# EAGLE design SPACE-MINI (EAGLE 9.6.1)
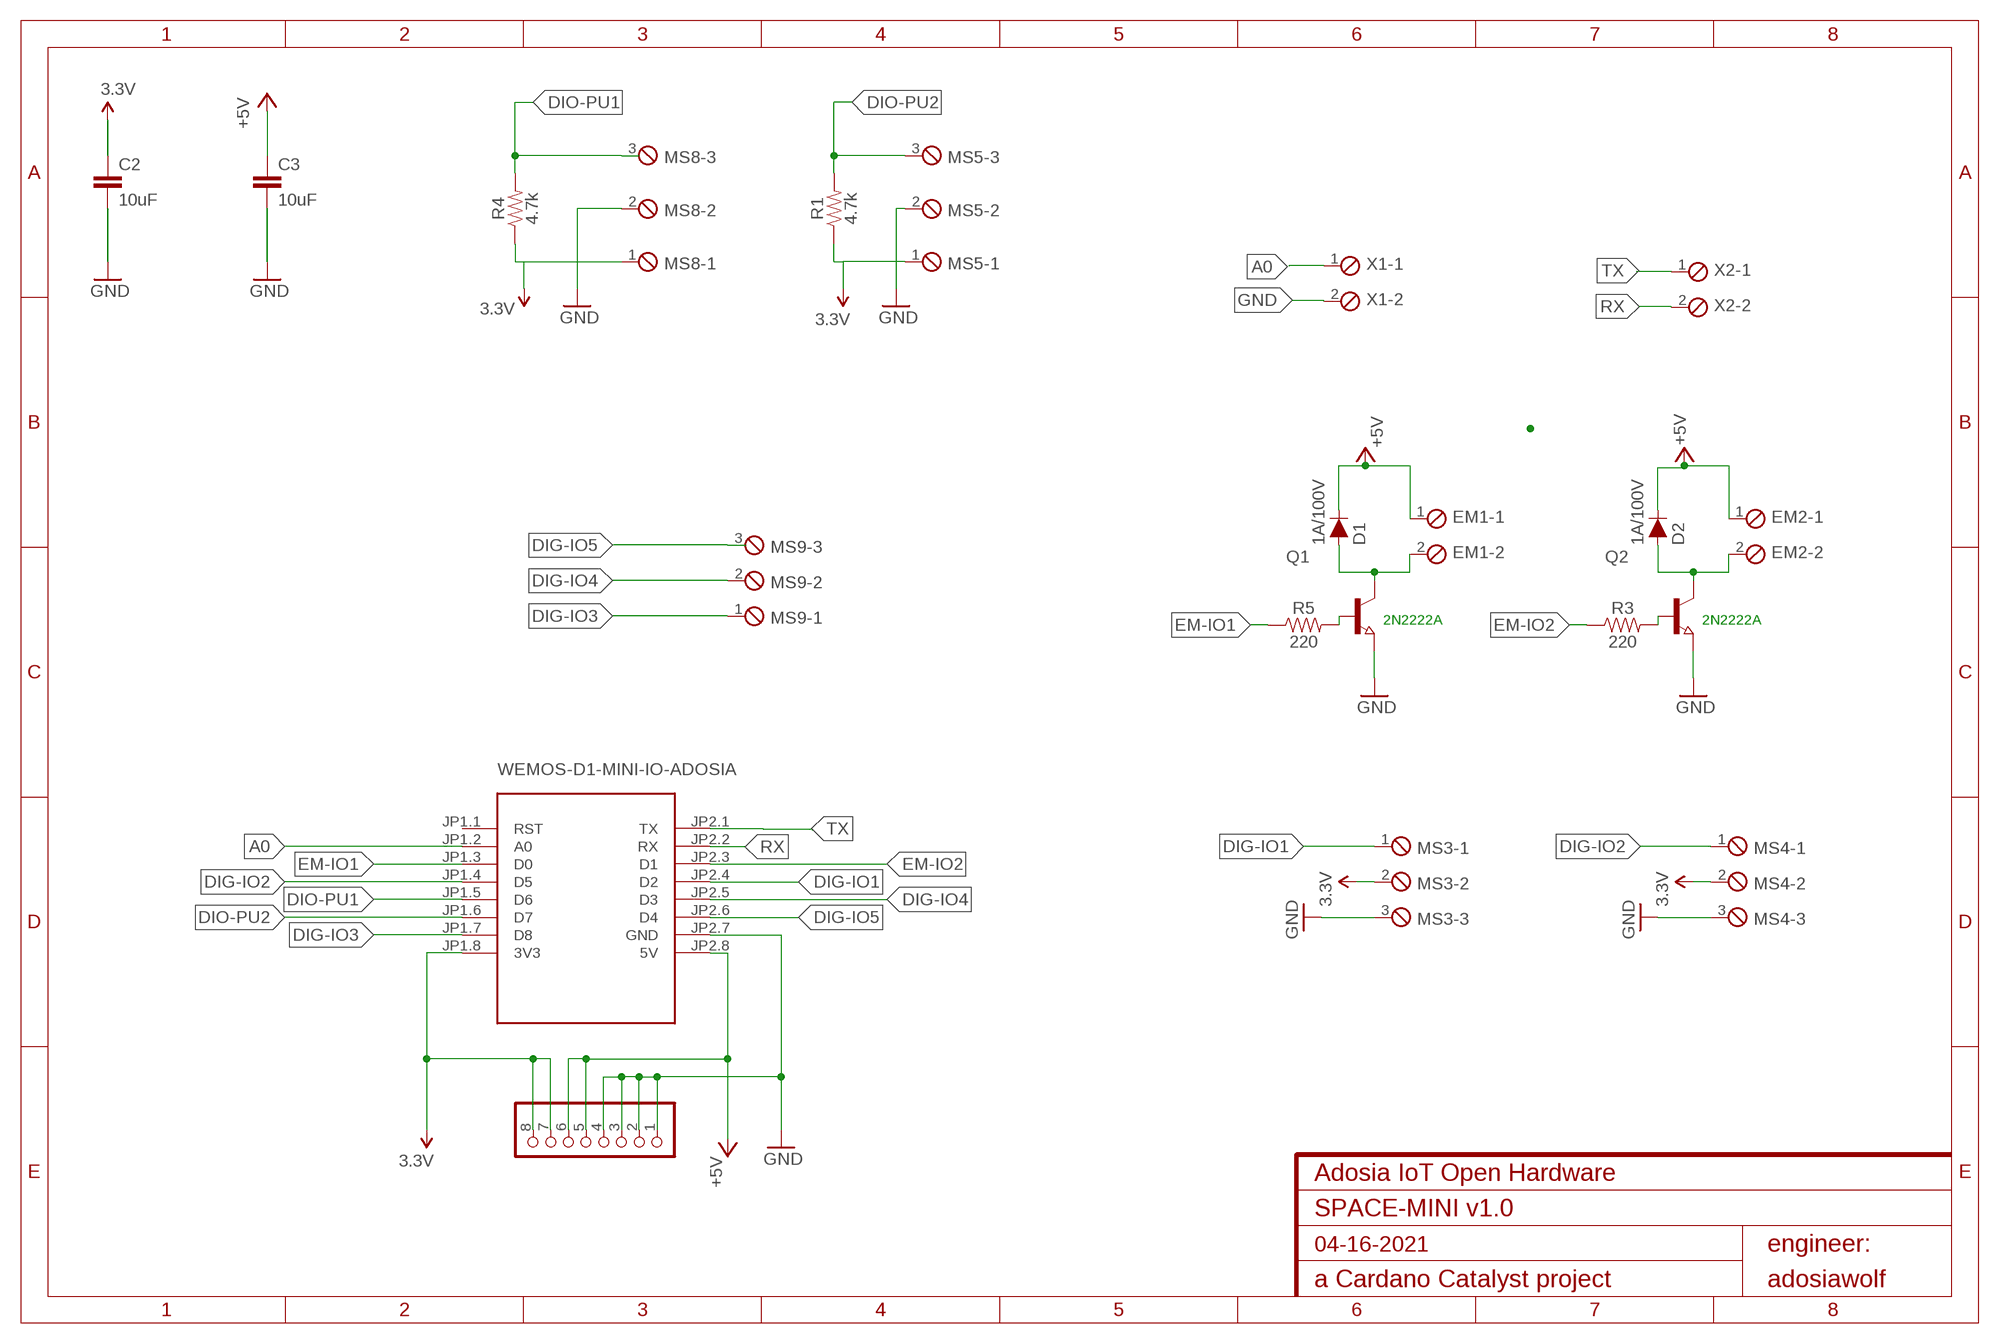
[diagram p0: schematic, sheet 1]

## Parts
C2  10uF  10UF-6.3V-20%(0603)  [0603-CAP@1]
C3  10uF  10UF-6.3V-20%(0603)  [0603-CAP@1]
D1  1A/100V  DIODE-BAS16J  [SOD-323]
D2  1A/100V  DIODE-BAS16J  [SOD-323]
EM1  MPT2  [2POL254]
EM2  MPT2  [2POL254]
JP1  PINHD-1X8/90  [1X08/90]
MS3  MPT3  [3POL254]
MS4  MPT3  [3POL254]
MS5  MPT3  [3POL254]
MS8  MPT3  [3POL254]
MS9  MPT3  [3POL254]
Q1  NPN-TRANSISTOR_SOT23  [SOT23]
Q2  NPN-TRANSISTOR_SOT23  [SOT23]
R1  4.7k  4.7KOHM-0603-1/10W-1%  [0603]
R3  220  220OHM-0603-1/10W-1%  [0603]
R4  4.7k  4.7KOHM-0603-1/10W-1%  [0603]
R5  220  220OHM-0603-1/10W-1%  [0603]
U$1  WEMOS-D1-MINI-IO-ADOSIA  [WEMOS-D1-MINI-SHIELD]
X1  MPT2  [2POL254]
X2  MPT2  [2POL254]

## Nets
3.3V: C2.1 JP1.7 JP1.8 MS3.2 MS4.2 MS5.1 MS8.1 R1.1 R4.1 U$1.JP1.8(3V3)
+5V: C3.1 D1.C D2.C EM1.1 EM2.1 JP1.5 JP1.6 U$1.JP2.8(5V)
A0: U$1.JP1.2(A0) X1.1
DIG-IO1: MS3.1 U$1.JP2.4(D2)
DIG-IO2: MS4.1 U$1.JP1.4(D5)
DIG-IO3: MS9.1 U$1.JP1.7(D8)
DIG-IO4: MS9.2 U$1.JP2.5(D3)
DIG-IO5: MS9.3 U$1.JP2.6(D4)
DIO-PU1: MS8.3 R4.2 U$1.JP1.5(D6)
DIO-PU2: MS5.3 R1.2 U$1.JP1.6(D7)
EM-IO1: R5.1 U$1.JP1.3(D0)
EM-IO2: R3.1 U$1.JP2.3(D1)
GND: C2.2 C3.2 JP1.1 JP1.2 JP1.3 JP1.4 MS3.3 MS4.3 MS5.2 MS8.2 Q1.2(E) Q2.2(E) U$1.JP2.7(GND) X1.2
N$2: Q2.1(B) R3.2
N$3: Q1.1(B) R5.2
N$4: D2.A EM2.2 Q2.3(C)
N$6: D1.A EM1.2 Q1.3(C)
RX: U$1.JP2.2(RX) X2.2
TX: U$1.JP2.1(TX) X2.1
Unconnected: U$1.JP1.1(RST)

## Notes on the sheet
- 2N2222A | 2N2222A

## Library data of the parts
C2 C3 = SparkFun-Capacitors:10UF-6.3V-20%(0603): CAP-11015; PROD_ID: CAP-11015
D1 D2 = SparkFun-DiscreteSemi:DIODE: Diode; PROD_ID: DIO-09646; VALUE: 250mA/100V
EM1 EM2 X1 X2 = con-phoenix-254:MPT2: PHOENIX CONNECTOR; OC_FARNELL: unknown; OC_NEWARK: unknown
JP1 = pinhead:PINHD-1X8: PIN HEADER
MS3-MS5 MS8 MS9 = con-phoenix-254:MPT3: PHOENIX CONNECTOR; OC_FARNELL: unknown; OC_NEWARK: unknown
Q1 Q2 = semicon-smd-ipc:NPN-TRANSISTOR_: NPN TRANSISTOR
R1 R4 = SparkFun-Resistors:4.7KOHM: 4.7kΩ resistor; PROD_ID: RES-07857
R3 R5 = SparkFun-Resistors:220OHM: 220Ω resistor; PROD_ID: RES-07861
U$1 = diy-modules:WEMOS-D1-MINI-IO-ADOSIA: Template for WEMOS D1 mini compatible shields NOTICE: This is a template only. You can use it as a base to create symbols for WEMOS D1 mini compatible shields. Official list of available shields can be found here: https://www.wemos.cc/D1-mini-Shields

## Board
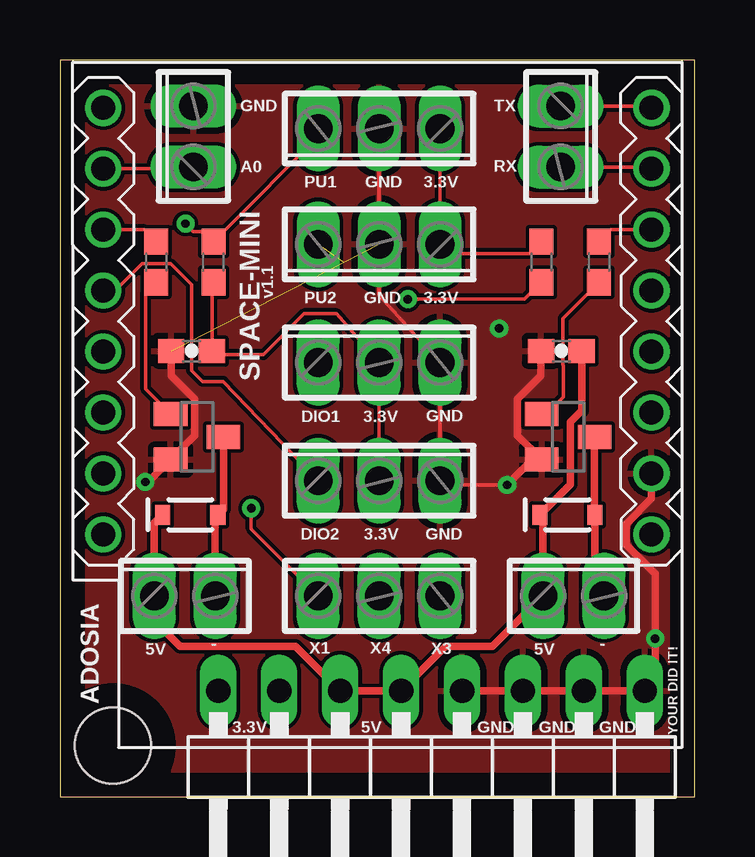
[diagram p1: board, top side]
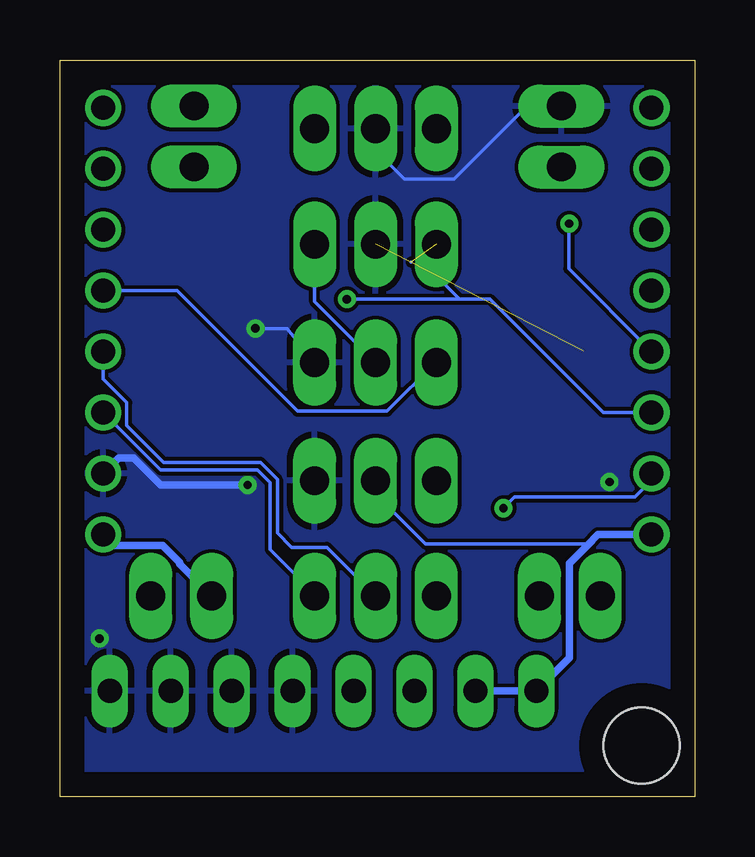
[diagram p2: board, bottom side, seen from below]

Size 26.47 x 30.72 mm. Coordinates in mm from the lower left corner, seen from the top.
Outline: 0,0 26.47,0 26.47,30.72 0,30.72 0,0
Copper layers (1*16): Top 0.035mm / dielectric 1.5mm / Bottom 0.035mm
Design rules "default": minimum track width 6mil, minimum drill 0.35mm, track to track 6mil, track to pad 6mil, pad to pad 6mil, via to via 6mil, smd to smd 6mil, copper to edge 40mil, drill to drill 6mil, minimum pad ring 10mil, minimum via ring 8mil, stop-mask expansion 4mil, vias tented up to drill 0mil, thermal gap 10mil
Holes 3.17 mm at 2.21,2.13

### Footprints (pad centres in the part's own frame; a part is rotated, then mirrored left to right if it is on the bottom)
0603-CAP@1 = smd 1.1 x 1: 1 -0.85,0; 2 0.85,0
SOD-323 = smd 0.63 x 0.83: A 1.15,0; C -1.15,0
2POL254 = drill 1.2 long: 1 -1.27,0; 2 1.27,0
1X08/90 = drill 1.016 long: 1 -8.89,-3.81; 2 -6.35,-3.81; 3 -3.81,-3.81; 4 -1.27,-3.81; 5 1.27,-3.81; 6 3.81,-3.81; 7 6.35,-3.81; 8 8.89,-3.81
3POL254 = drill 1.2 long: 1 -2.54,0; 2 0,0; 3 2.54,0
SOT23 = smd 1 x 1.4: 1 -0.95,-1.1; 2 0.95,-1.1; 3 0,1.1
0603 = smd 1.1 x 1: 1 -0.85,0; 2 0.85,0
WEMOS-D1-MINI-SHIELD = drill 1: JP1.1 -11.43,12.065; JP1.2 -11.43,9.525; JP1.3 -11.43,6.985; JP1.4 -11.43,4.445; JP1.5 -11.43,1.905; JP1.6 -11.43,-0.635; JP1.7 -11.43,-3.175; JP1.8 -11.43,-5.715; JP2.1 11.43,12.065; JP2.2 11.43,9.525; JP2.3 11.43,6.985; JP2.4 11.43,4.445; JP2.5 11.43,1.905; JP2.6 11.43,-0.635; JP2.7 11.43,-3.175; JP2.8 11.43,-5.715

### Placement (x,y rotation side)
C2  5.49,18.59 180 top
C3  20.9,18.59 180 top
D1  5.44,11.76 0 top
D2  21.16,11.76 0 top
EM1  5.21,8.38 0 top
EM2  21.41,8.38 0 top
JP1  15.49,0.61 180 top
MS3  13.31,18.11 0 top
MS4  13.31,13.18 0 top
MS5  13.31,23.04 180 top
MS8  13.31,27.86 180 top
MS9  13.31,8.38 0 top
Q1  5.71,15.01 270 top
Q2  21.18,15.01 270 top
R1  20.07,22.3 270 top
R3  22.48,22.3 270 top
R4  6.4,22.3 90 top
R5  4.01,22.3 270 top
U$1  13.23,16.66 0 top
X1  5.56,27.53 90 top
X2  20.88,27.53 270 top

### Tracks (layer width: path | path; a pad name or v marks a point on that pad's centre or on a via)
3.3V
  Top 0.152: R4.1 6.34,21.39 C2.1 6.49,18.44 8.48,18.44 10.19,20.14 11.53,20.14 MS3.2 MS4.2 | MS8.1 MS5.1 16.51,22.66 19.57,22.66 R1.1
  Bottom 0.152: JP1.7 9.45,4.42 | MS5.1 15.85,20.65 MS3.2 | MS4.2 13.31,12.62 11.23,10.54 4.5,10.54 4.46,10.51
  Bottom 0.305: U$1.JP1.8 2.39,10.95 2.39,10.94 4.03,10.94 4.46,10.51 5.23,9.74 5.23,5.79 JP1.8 JP1.7
+5V
  Top 0.305: D1.C 3.94,11.41 EM1.1 3.94,7.34 5,6.27 9.83,6.27 JP1.6 JP1.5 16.08,6.28 18.04,6.28 EM2.1 20.14,11.63 D2.C 21.28,13.03 21.28,15.64 21.75,16.11 C3.1
  Bottom 0.305: U$1.JP2.8 24.2,10.49 22.18,10.49 21.48,9.78 21.48,9.72 EM2.1
A0
  Top 0.152: U$1.JP1.2 5.49,26.19 X1.1
DIG-IO1
  Bottom 0.152: U$1.JP2.4 21.59,21.11 16.56,16.08 12.83,16.08 10.77,18.14 MS3.1
DIG-IO2
  Top 0.152: MS4.1 6.81,17.32 5.94,17.32 5.49,17.78 5.49,21.35 4.61,22.23 3.42,22.23 2.3,21.11 U$1.JP1.4
DIG-IO3  (via drill 0.35)
  Top 0.152: MS9.1 7.98,11.18 v7.98,12.04
  Bottom 0.152: v7.98,12.04 7.52,12.5 2.49,12.5 1.8,13.18 U$1.JP1.7
DIG-IO4
  Bottom 0.152: U$1.JP2.5 24.66,17.42 23.68,16.43 23.68,15.48 22.15,13.94 18.11,13.94 17.4,13.23 17.4,11 16.81,10.41 15.34,10.41 MS9.2
DIG-IO5
  Bottom 0.152: U$1.JP2.6 22.28,13.64 18.24,13.64 17.7,13.11 17.7,10.31 15.85,8.46 MS9.3
DIO-PU1  (via drill 0.35)
  Top 0.152: R4.2 6.83,23.58 | 6.83,23.58 10.77,27.52 MS8.3 | v5.23,23.9 5.56,23.58 6.83,23.58
  Bottom 0.152: U$1.JP1.5 5.26,22.02 5.26,23.88 v5.23,23.9
DIO-PU2  (via drill 0.35)  (1 unrouted)
  Top 0.152: R1.2 19.37,20.76 v14.51,20.76 v14.5,20.75
  Bottom 0.152: U$1.JP1.6 3.81,16.03 8.53,20.75 9.8,20.75 | 11.82,22.31 11.82,22.29 | v14.5,20.75 9.8,20.75 | MS5.3 10.77,21.72 9.8,20.75
EM-IO1
  Top 0.152: R5.1 3.52,23.65 U$1.JP1.3
EM-IO2
  Top 0.152: R3.1 22.98,23.65 U$1.JP2.3
GND  (via drill 0.35)  (1 unrouted)
  Top 0.152: v18.64,13.01 16.2,13.01 MS4.3 MS3.3 13.31,20.93 MS5.2 MS8.2
  Top 0.305: C3.2 20.05,17.56 19.08,16.59 19.08,15.07 Q2.2 19.7,14.06 v18.64,13.01 | C2.2 4.64,17.57 5.62,16.59 5.62,15.07 Q1.2 3.69,13.13 v3.56,13.13 | U$1.JP2.7 24.66,12.45 23.61,11.39 23.61,10.51 24.82,9.3 v24.82,6.6 24.82,4.85 JP1.1 JP1.2 JP1.3 JP1.4
  Bottom 0.152: X1.2 7,28.8 10.05,25.76 12.09,25.76 13.29,26.96 13.29,27.88 MS8.2 | v18.31,19.53 16.99,19.53 MS3.3
  Bottom 0.305: v18.64,13.01 22.28,13.01 23.39,14.12 24.03,14.12 U$1.JP2.7
  pour Bottom: -0.2,30.86 -0.2,-0.28 26.67,-0.28 26.67,30.86
  pour Top: -0.2,30.86 -0.2,-0.28 26.67,-0.28 26.67,30.86
N$2
  Top 0.152: R3.2 20.98,19.95 20.98,18 20.98,17.99 20.98,16.66 20.28,15.96 Q2.1
N$3
  Top 0.152: Q1.1 3.58,17 3.58,21.02 R5.2
N$4
  Top 0.305: Q2.3 22.28,11.79 D2.A 22.31,8.76 EM2.2
N$6
  Top 0.305: Q1.3 6.82,11.99 D1.A 6.48,11.65 EM1.2
RX
  Top 0.152: X2.2 24.59,26.26 U$1.JP2.2
TX
  Top 0.152: X2.1 24.59,28.8 U$1.JP2.1

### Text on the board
tNames: GND | TX | A0 | PU1 | GND | 3.3V | RX | SPACE-MINI | v1.1 | PU2 | GND | 3.3V | DIO1 | 3.3V | GND | DIO2 | 3.3V | GND | ADOSIA | 5V | - | X1 | X4 | X3 | 5V | - | YOUR DID IT! | 3.3V | 5V | GND | GND | GND

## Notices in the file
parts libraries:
SparkFun-Aesthetics: Licensing: CC v3.0 Share-Alike You are welcome to use this library for commercial purposes.
SparkFun-Capacitors: Licensing: Creative Commons ShareAlike 4.0 International - https://creativecommons.org/licenses/by-sa/4.0
